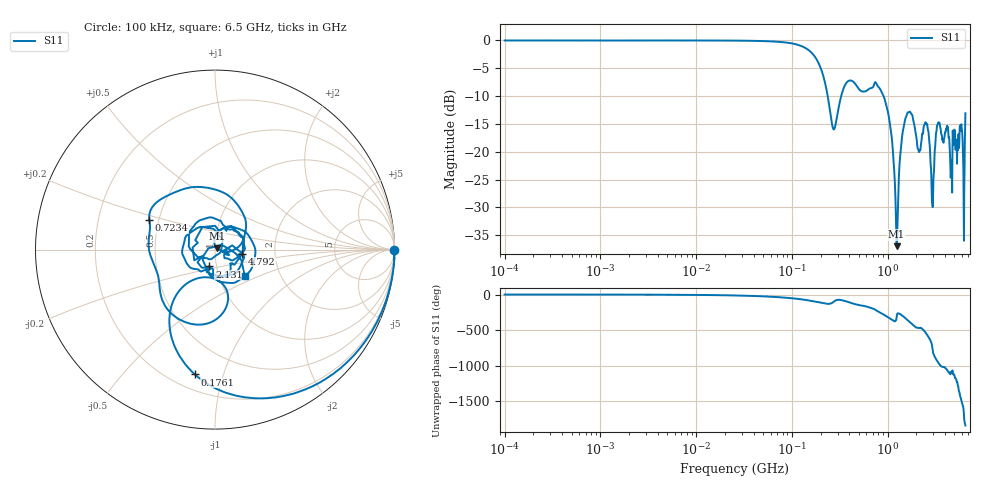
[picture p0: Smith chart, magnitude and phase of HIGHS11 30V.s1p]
!Keysight Technologies,E5080B,MY59100498,A.17.05.10
!Date: Wednesday, August 30, 2023 19:25:22
!Correction: S11(C  1-Port  )
!S1P File: Measurement: S11:Log Frequency Sweep
# Hz S  dB  R 50
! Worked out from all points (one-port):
!   1601 points, 100 kHz to 6.5 GHz, reference 50 ohm
!   lowest |S11| = -37.0 dB at 1.242 GHz (marker M1), VSWR 1.03, Z = 51.2 + j0.848 ohm
!   |S11| at or under -10 dB: 236.9 MHz to 327.8 MHz (90.87 MHz wide, 32.2 % of centre); 907.9 MHz to end of sweep
!   S11 on the Smith chart (normalised r, x): 100 kHz: open; 176.1 MHz: 0.29, -0.81; 723.4 MHz: 0.44, +0.17; 2.131 GHz: 0.92, -0.18; 4.792 GHz: 1.36, -0.06; 6.5 GHz: 1.32, -0.41
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100000  -0.00 -0.1
399589.6  -0.00 -0.2
1596718  -0.01 -0.8
6380321  -0.00 -3.2
2.54951e7  -0.03 -12.7
5.894314e7  -0.15 -29.9
1.018758e8  -0.55 -53.3
1.401013e8  -1.40 -76.2
1.760794e8  -3.05 -99.1
2.182522e8  -7.06 -124.7
2.724062e8  -15.96 -103.2
3.28424e8  -9.95 -78.1
4.070849e8  -7.19 -114.0
7.233607e8  -7.94 156.0
8.482825e8  -8.94 102.5
1.022724e9  -13.34 36.4
1.241608e9  -36.99 35.9
1.416243e9  -17.36 65.6
1.626669e9  -12.93 -2.1
1.817307e9  -13.51 -61.9
2.13115e9  -20.08 -108.2
2.551666e9  -15.07 164.7
2.930793e9  -29.33 -25.6
3.389649e9  -14.76 121.4
4.172505e9  -15.33 21.7
4.792457e9  -16.21 -8.2
5.317155e9  -22.16 -153.2
6.5e9  -13.09 -41.6
